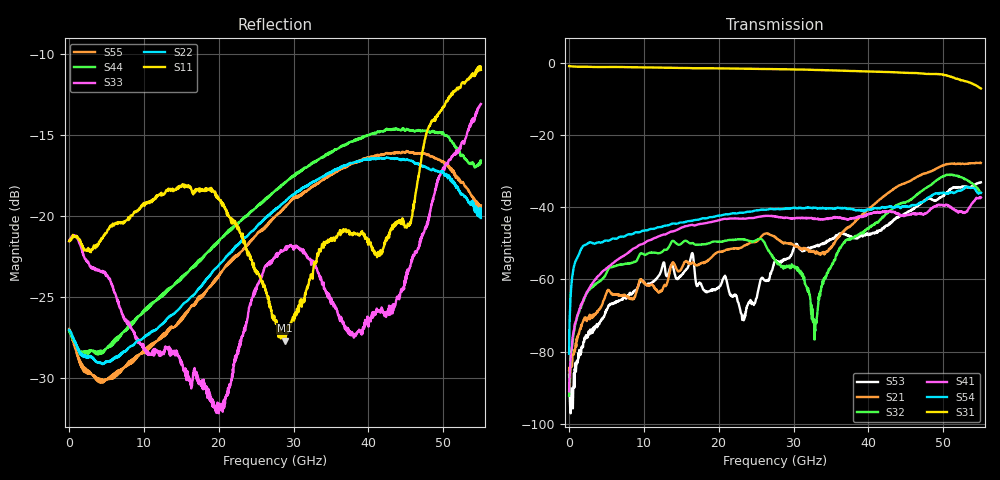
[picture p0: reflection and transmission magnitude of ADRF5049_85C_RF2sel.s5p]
! Device  : ADRF5049
! Description: Silicon SP4T Switch Non-Reflective
! Frequency:  9kHz -  45 GHz
! Ports:
!  RFC = Port 1
!  RF1 = Port 2
!  RF2 = Port 3
!	 RF3 = Port 4
!  RF4 = Port 5
! VSS  =  +3.30 Volts
! VDD  =  -3.30 Volts
! EN  =  0.00 Volts
! LS  =  0.00 Volts
! V1  =  3.30 Volts
! V2  =  0.00 Volts
! Data:  Data was collected using an calibrated 4 port network analyzer.
! Notes: Analog Devices supplies this data as a sample of measured data
!  for this product.  Your particular data for this product may vary.
!  Data was taken at 85 degrees C.
!  Analog Devices reserves the right to change this data at anytime.
# hz S db R 50
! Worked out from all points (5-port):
!   1100 points, 50 MHz to 55 GHz, reference 50 ohm
!   strongest paths, dB at 50 MHz, 13.8 GHz, 27.55 GHz, 41.3 GHz, 55 GHz:
!     S31: -0.8, -1.3, -1.6, -2.4, -7.0
!     S54: -80.6, -44.5, -40.5, -40.2, -36.0
!     S41: -91.0, -46.7, -42.5, -41.3, -37.3
!     S32: -92.2, -49.4, -54.7, -44.0, -35.9
!     S21: -85.2, -55.5, -48.2, -38.2, -27.7
!     S53: -86.5, -56.0, -54.8, -46.7, -33.1
!   lowest |S11| = -27.7 dB at 28.85 GHz (marker M1), VSWR 1.09, Z = 51.2 - j4.02 ohm
!   |S11| at or under -10 dB: start of sweep to end of sweep
